| IBIS file usslh4gxxac.ibs
| 4Gb DDR3L SDRAM - Die Revision "D"
| This Model is valid for Commercial Temperature Range -40C<=Tc<=95C
| Valid for DDR3L-1066/1333/1600/1866/2133 operation
| Part Number   VDD/VDDQ   Architecture   Package
| SCB13H4G800AF   1.35V/1.35V   512Meg x 8   78-Ball 7.5x10.6mm FBGA
| SCB13H4G800AF KGD 1.35V/1.35V   512Meg x 8   Bare Die
| SCB13H4G160AF   1.35V/1.35V   256Meg x 16  96-Ball 7.5x13.5mm FBGA
| SCB13H4G160AF KGD 1.35V/1.35V   256Meg x 16  Bare Die
[IBIS Ver]   4.2
[File Name]   usslh4gxxac.ibs
[Date]   12/20/2020
[File Rev]   1.2
[Source]   UniIC
[Notes]   Revision History:
   Rev 1.0: 01/23/2019
   - For VDD1.50V
   Rev 1.1: 12/12/2019
   - Change VDD level to 1.35V from 1.50V
   Rev 1.2: 12/20/2020
   - Change temp to -40C from 0C
   - update 95c data
[Disclaimer]  --
[Copyright]   Copyright 2020. UniIC All rights reserved.
| COMPONENT: SCB13H4G800AF (78-Ball FBGA, x8, 7.5mm X 10.6mm)
[Component]   SCB13H4G800AF
[Package Model] f25_4gd3_x8_78ball_pkg
[Manufacturer]  UniIC.
[Package]
|   typ   min   max
R_pkg   404m   282m   555m
L_pkg   1.730nH   1.139nH   2.492nH
C_pkg   0.438pF   0.389pF   0.762pF
[Pin]   signal_name  model_name   R_pin  L_pin   C_pin
A1   VSS   GND
A2   VDD   POWER
A3   NC   NC
A7   NF_TDQS#   NF_TDQS#   474m   1.870nH   0.560pF
A8   VSS   GND
A9   VDD   POWER
B1   VSS   GND
B2   VSSQ   GND
B3   DQ0   DQ   499m   1.667nH   0.564pF
B7   DM_TDQS   DM_TDQS   474m   1.582nH   0.537pF
B8   VSSQ   GND
B9   VDDQ   POWER
C1   VDDQ   POWER
C2   DQ2   DQ   555m   2.075nH   0.595pF
C3   DQS   DQS   476m   1.795nH   0.574pF
C7   DQ1   DQ   401m   1.399nH   0.540pF
C8   DQ3   DQ   504m   1.705nH   0.567pF
C9   VSSQ   GND
D1   VSSQ   GND
D2   DQ6   DQ   504m   1.669nH   0.567pF
D3   DQS#   DQS   480m   1.782nH   0.568pF
D7   VDD   POWER
D8   VSS   GND
D9   VSSQ   GND
E1   VREFDQ   POWER
E2   VDDQ   POWER
E3   DQ4   DQ   399m   1.300nH   0.528pF
E7   DQ7   DQ   393m   1.400nH   0.549pF
E8   DQ5   DQ   472m   1.522nH   0.557pF
E9   VDDQ   POWER
F1   NC   NC
F2   VSS   GND
F3   RAS#   INPUT   367m   1.644nH   0.431pF
F7   CK   CLKIN   346m   1.230nH   0.390pF
F8   VSS   GND
F9   NC   NC
G1   ODT   INPUT   496m   2.492nH   0.516pF
G2   VDD   POWER
G3   CAS#   INPUT   397m   1.998nH   0.417pF
G7   CK#   CLKIN   349m   1.428nH   0.397pF
G8   VDD   POWER
G9   CKE   INPUT   432m   2.140nH   0.438pF
H1   NC   NC
H2   CS#   INPUT   376m   1.890nH   0.414pF
H3   WE#   INPUT   397m   1.729nH   0.41pF
H7   A10   INPUT   306m   1.139nH   0.402pF
H8   ZQ   NC   394m   1.459nH   0.417pF
H9   NC   NC
J1   VSS   GND
J2   BA0   INPUT   379m   1.786nH   0.401pF
J3   BA2   INPUT   446m   1.959nH   0.417pF
J7   A15   INPUT   282m   1.236nH   0.413pF
J8   VREFCA   POWER
J9   VSS   GND
K1   VDD   POWER
K2   A3   INPUT   404m   1.842nH   0.427pF
K3   A0   INPUT   323m   1.426nH   0.396pF
K7   A12   INPUT   319m   1.369nH   0.389pF
K8   BA1   INPUT   418m   1.866nH   0.445pF
K9   VDD   POWER
L1   VSS   GND
L2   A5   INPUT   394m   1.951nH   0.419pF
L3   A2   INPUT   336m   1.617nH   0.394pF
L7   A1   INPUT   310m   1.445nH   0.433pF
L8   A4   INPUT   405m   1.730nH   0.422pF
L9   VSS   GND
M1   VDD   POWER
M2   A7   INPUT   426m   2.163nH   0.456pF
M3   A9   INPUT   367m   1.851nH   0.433pF
M7   A11   INPUT   389m   1.709nH   0.415pF
M8   A6   INPUT   442m   2.110nH   0.458pF
M9   VDD   POWER
N1   VSS   GND
N2   RESET#   RESET   542m   1.964nH   0.762pF
N3   A13   INPUT   424m   2.205nH   0.441pF
N7   A14   INPUT   446m   1.873nH   0.447pF
N8   A8   INPUT   493m   2.378nH   0.503pF
N9   VSS   GND
|***********************PIN MAPPING*****************************************
[Pin Mapping] pulldown_ref pullup_ref gnd_clamp_ref power_clamp_ref ext_ref
A1   VSS   NC
A2   NC   VDD
A3   NC   NC
A7   VSS   VDDQ   VSS   VDDQ
A8   VSS   NC
A9   NC   VDD
B1   VSS   NC
B2   VSS   NC
B3   VSS   VDDQ   VSS   VDDQ
B7   VSS   VDDQ   VSS   VDDQ
B8   VSS   NC
B9   NC   VDDQ
C1   NC   VDDQ
C2   VSS   VDDQ   VSS   VDDQ
C3   VSS   VDDQ   VSS   VDDQ
C7   VSS   VDDQ   VSS   VDDQ
C8   VSS   VDDQ   VSS   VDDQ
C9   VSS   NC
D1   VSS   NC
D2   VSS   VDDQ   VSS   VDDQ
D3   VSS   VDDQ   VSS   VDDQ
D7   NC   VDD
D8   VSS   NC
D9   VSS   NC
E1   NC   VREFDQ
E2   NC   VDDQ
E3   VSS   VDDQ   VSS   VDDQ
E7   VSS   VDDQ   VSS   VDDQ
E8   VSS   VDDQ   VSS   VDDQ
E9   NC   VDDQ
F1   NC   NC
F2   VSSL   NC
F3   NC   NC   VSS   VDD
F7   NC   NC   VSS   VDD
F8   VSS   NC
F9   NC   NC
G1   NC   NC   VSS   VDD
G2   NC   VDDL
G3   NC   NC   VSS   VDD
G7   NC   NC   VSS   VDD
G8   NC   VDD
G9   NC   NC   VSS   VDD
H1   NC   NC
H2   NC   NC   VSS   VDD
H3   NC   NC   VSS   VDD
H7   NC   NC   VSS   VDD
H8   NC   NC
H9   NC   NC
J1   VSS   NC
J2   NC   NC   VSS   VDD
J3   NC   NC   VSS   VDD
J7   NC   NC   VSS   VDD
J8   NC   VREFCA
J9   VSS   NC
K1   NC   VDD
K2   NC   NC   VSS   VDD
K3   NC   NC   VSS   VDD
K7   NC   NC   VSS   VDD
K8   NC   NC   VSS   VDD
K9   NC   VDD
L1   VSS   NC
L2   NC   NC   VSS   VDD
L3   NC   NC   VSS   VDD
L7   NC   NC   VSS   VDD
L8   NC   NC   VSS   VDD
L9   VSS   NC
M1   NC   VDD
M2   NC   NC   VSS   VDD
M3   NC   NC   VSS   VDD
M7   NC   NC   VSS   VDD
M8   NC   NC   VSS   VDD
M9   NC   VDD
N1   VSS   NC
N2   NC   NC   VSS   VDD
N3   NC   NC   VSS   VDD
N7   NC   NC   VSS   VDD
N8   NC   NC   VSS   VDD
N9   VSS   NC
|**********************DIFF PIN*********************************************
[Diff_pin]   inv_pin   vdiff   tdelay_typ   tdelay_min   tdelay_max
   C3   D3   0.320V   0ns   NA   NA
   F7   G7   0.320V   0ns   NA   NA
| COMPONENT: SCB13H4G160AF (96-Ball FBGA, x16, 7.5mm X 13.5mm)
[Component]   SCB13H4G160AF
[Package Model] f25_4gd3_x16_96ball_pkg
[Manufacturer]  UniIC.
[Package]
|   typ   min   max
R_pkg   449m   320m   623m
L_pkg   1.828nH   1.147nH   3.053nH
C_pkg   0.538pF   0.376pF   0.812pF
[Pin]   signal_name  model_name   R_pin   L_pin   C_pin
A1   VDDQ   POWER
A2   DQ13   DQ   581m   2.212nH  0.592pF
A3   DQ15   DQ   536m   1.891nH  0.554pF
A7   DQ12   DQ   536m   1.903nH  0.565pF
A8   VDDQ   POWER
A9   VSS   GND
B1   VSSQ   GND
B2   VDD   POWER
B3   VSS   GND
B7   UDQS#   DQS   503m   1.737nH  0.583pF
B8   DQ14   DQ   582m   2.266nH  0.574pF
B9   VSSQ   GND
C1   VDDQ   POWER
C2   DQ11   DQ   488m   1.893nH  0.538pF
C3   DQ9   DQ   421m   1.377nH  0.561pF
C7   UDQS   DQS   507m   1.684nH  0.57pF
C8   DQ10   DQ   562m   2.137nH  0.556pF
C9   VDDQ   POWER
D1   VSSQ   GND
D2   VDDQ   POWER
D3   UDM   DM   424m   1.243nH  0.563pF
D7   DQ8   DQ   367m   1.215nH  0.531pF
D8   VSSQ   GND
D9   VDD   POWER
E1   VSS   GND
E2   VSSQ   GND
E3   DQ0   DQ   385m   1.248nH  0.558pF
E7   LDM   DM   384m   1.183nH  0.556pF
E8   VSSQ   GND
E9   VDDQ   POWER
F1   VDDQ   POWER
F2   DQ2   DQ   486m   1.450nH  0.569pF
F3   LDQS   DQS   441m   1.603nH  0.55pF
F7   DQ1   DQ   358m   1.147nH  0.544pF
F8   DQ3   DQ   454m   1.411nH  0.551pF
F9   VSSQ   GND
G1   VSSQ   GND
G2   DQ6   DQ   440m   1.316nH  0.541pF
G3   LDQS#   DQS   438m   1.640nH  0.542pF
G7   VDD   POWER
G8   VSS   GND
G9   VSSQ   GND
H1   VREFDQ   POWER
H2   VDDQ   POWER
H3   DQ4   DQ   402m   1.262nH  0.562pF
H7   DQ7   DQ   415m   1.353nH  0.563pF
H8   DQ5   DQ   544m   1.670nH  0.569pF
H9   VDDQ   POWER
J1   NC   NC
J2   VSS   GND
J3   RAS#   INPUT   320m   1.391nH  0.443pF
J7   CK   CLKIN   335m   1.168nH  0.376pF
J8   VSS   GND
J9   NC   NC
K1   ODT   INPUT   449m   2.344nH  0.449pF
K2   VDD   POWER
K3   CAS#   INPUT   328m   1.520nH  0.451pF
K7   CK#   CLKIN   327m   1.315nH  0.387pF
K8   VDD   POWER
K9   CKE   INPUT   496m   2.272nH  0.497pF
L1   NC   NC
L2   CS#   INPUT   414m   2.027nH  0.446pF
L3   WE#   INPUT   349m   1.670nH  0.436pF
L7   A10   INPUT   350m   1.335nH  0.447pF
L8   ZQ   NC   479m   1.675nH  0.492pF
L9   NC   NC
M1   VSS   GND
M2   BA0   INPUT   430m   2.210nH  0.443pF
M3   BA2   INPUT   400m   1.828nH  0.449pF
M7   NC   NC
M8   VREFCA   POWER
M9   VSS   GND
N1   VDD   POWER
N2   A3   INPUT   488m   2.298nH  0.493pF
N3   A0   INPUT   392m   1.664nH  0.456pF
N7   A12   INPUT   382m   1.894nH  0.476pF
N8   BA1   INPUT   484m   2.159nH  0.499pF
N9   VDD   POWER
P1   VSS   GND
P2   A5   INPUT   515m   2.412nH  0.524pF
P3   A2   INPUT   447m   2.102nH  0.537pF
P7   A1   INPUT   415m   2.085nH  0.516pF
P8   A4   INPUT   498m   2.422nH  0.534pF
P9   VSS   GND
R1   VDD   POWER
R2   A7   INPUT   565m   2.745nH  0.585pF
R3   A9   INPUT   492m   2.376nH  0.531pF
R7   A11   INPUT   452m   2.341nH  0.506pF
R8   A6   INPUT   559m   2.746nH  0.595pF
R9   VDD   POWER
T1   VSS   GND
T2   RESET#   RESET   623m   2.039nH  0.812pF
T3   A13   INPUT   556m   2.572nH  0.547pF
T7   A14   INPUT   518m   2.557nH  0.521pF
T8   A8   INPUT   583m   3.053nH  0.578pF
T9   VSS   GND
|***********************PIN MAPPING*****************************************
[Pin Mapping] pulldown_ref pullup_ref gnd_clamp_ref power_clamp_ref ext_ref
A1   NC   VDDQ
A2   VSS   VDDQ   VSS   VDDQ
A3   VSS   VDDQ   VSS   VDDQ
A7   VSS   VDDQ   VSS   VDDQ
A8   NC   VDDQ
A9   VSS   NC
B1   VSS   NC
B2   NC   VDD
B3   VSS   NC
B7   VSS   VDDQ   VSS   VDDQ
B8   VSS   VDDQ   VSS   VDDQ
B9   VSS   NC
C1   NC   VDDQ
C2   VSS   VDDQ   VSS   VDDQ
C3   VSS   VDDQ   VSS   VDDQ
C7   VSS   VDDQ   VSS   VDDQ
C8   VSS   VDDQ   VSS   VDDQ
C9   NC   VDDQ
D1   VSS   NC
D2   NC   VDDQ
D3   NC   NC   VSS   VDDQ
D7   VSS   VDDQ   VSS   VDDQ
D8   VSS   NC
D9   NC   VDD
E1   VSS   NC
E2   VSS   NC
E3   VSS   VDDQ   VSS   VDDQ
E7   NC   NC   VSS   VDDQ
E8   VSS   NC
E9   NC   VDDQ
F1   NC   VDDQ
F2   VSS   VDDQ   VSS   VDDQ
F3   VSS   VDDQ   VSS   VDDQ
F7   VSS   VDDQ   VSS   VDDQ
F8   VSS   VDDQ   VSS   VDDQ
F9   VSS   NC
G1   VSS   NC
G2   VSS   VDDQ   VSS   VDDQ
G3   VSS   VDDQ   VSS   VDDQ
G7   NC   VDD
G8   VSS   NC
G9   VSS   NC
H1   NC   VREFDQ
H2   NC   VDDQ
H3   VSS   VDDQ   VSS   VDDQ
H7   VSS   VDDQ   VSS   VDDQ
H8   VSS   VDDQ   VSS   VDDQ
H9   NC   VDDQ
J1   NC   NC
J2   VSSL   NC
J3   NC   NC   VSS   VDD
J7   NC   NC   VSS   VDD
J8   VSS   NC
J9   NC   NC
K1   NC   NC   VSS   VDD
K2   NC   VDDL
K3   NC   NC   VSS   VDD
K7   NC   NC   VSS   VDD
K8   NC   VDD
K9   NC   NC   VSS   VDD
L1   NC   NC
L2   NC   NC   VSS   VDD
L3   NC   NC   VSS   VDD
L7   NC   NC   VSS   VDD
L8   NC   NC
L9   NC   NC
M1   VSS   NC
M2   NC   NC   VSS   VDD
M3   NC   NC   VSS   VDD
M7   NC   NC
M8   NC   VREFCA
M9   VSS   NC
N1   NC   VDD
N2   NC   NC   VSS   VDD
N3   NC   NC   VSS   VDD
N7   NC   NC   VSS   VDD
N8   NC   NC   VSS   VDD
N9   NC   VDD
P1   VSS   NC
P2   NC   NC   VSS   VDD
P3   NC   NC   VSS   VDD
P7   NC   NC   VSS   VDD
P8   NC   NC   VSS   VDD
P9   VSS   NC
R1   NC   VDD
R2   NC   NC   VSS   VDD
R3   NC   NC   VSS   VDD
R7   NC   NC   VSS   VDD
R8   NC   NC   VSS   VDD
R9   NC   VDD
T1   VSS   NC
T2   NC   NC   VSS   VDD
T3   NC   NC   VSS   VDD
T7   NC   NC   VSS   VDD
T8   NC   NC   VSS   VDD
T9   VSS   NC
|**********************DIFF PIN*********************************************
[Diff_pin]   inv_pin   vdiff   tdelay_typ   tdelay_min   tdelay_max
   C7   B7   0.320V   0ns   NA   NA
   F3   G3   0.320V   0ns   NA   NA
   J7   K7   0.320V   0ns   NA   NA
| COMPONENT: SCB13H4G800AF KGD (Bare Die, x8)
[Component]   SCB13H4G800AF KGD
[Manufacturer]  UniIC.
[Package]
|   typ   min   max
R_pkg   0.001m   0.001m   0.001m
L_pkg   0.001nH   0.001nH   0.001nH
C_pkg   0.001pF   0.001pF   0.001pF
[Pin]   signal_name  model_name   R_pin   L_pin   C_pin
1   DNU   NC
2   VSS   GND
3   VDD   POWER
4   VDD   POWER
5   DNU   NC
6   VSS   GND
7   DNU   NC
8   VDDQ   POWER
9   DNU   NC
10   VSS   GND
11   DNU   NC
12   VDDQ   POWER
13   DNU   NC
14   VSS   GND
15   DNU   NC
16   DNU   NC
17   VDDQ   POWER
18   DNU   NC
19   VSS   GND
20   DNU   NC
21   VDDQ   POWER
22   DNU   NC
23   VSS   GND
24   DNU   NC
25   VDDQ   POWER
26   NF_TDQS#   NF_TDQS#
27   VSS   GND
28   VDD   POWER
29   VSS   GND
30   DM_TDQS   DM_TDQS
31   VDDQ   POWER
32   DQ0   DQ
33   VSS   GND
34   DQ1   DQ
35   VDDQ   POWER
36   DQ2   DQ
37   VSS   GND
38   DQ3   DQ
39   VDDQ   POWER
40   DQS   DQS
41   DQS#   DQS
42   VSS   GND
43   DQ6   DQ
44   VDDQ   POWER
45   DQ5   DQ
46   VSS   GND
47   DQ4   DQ
48   VDDQ   POWER
49   DQ7   DQ
50   VSS   GND
51   VREFDQ   POWER
52   VSS   GND
53   VDD   POWER
54   DNU   NC
55   VDD   POWER
56   VSS   GND
57   CK   CLKIN
58   CK#   CLKIN
59   CKE   INPUT
60   RAS#   INPUT
61   ODT   INPUT
62   CAS#   INPUT
63   CS#   INPUT
64   WE#   INPUT
65   A10   INPUT
66   VDD   POWER
67   VREFCA   POWER
68   VSS   GND
69   ZQ   NC
70   BA0   INPUT
71   BA1   INPUT
72   BA2   INPUT
73   A15   INPUT
74   A3   INPUT
75   A12   INPUT
76   VDD   POWER
77   VSS   GND
78   A0   INPUT
79   A4   INPUT
80   A5   INPUT
81   A6   INPUT
82   A2   INPUT
83   A1   INPUT
84   A7   INPUT
85   A8   INPUT
86   A9   INPUT
87   A11   INPUT
88   A13   INPUT
89   A14   INPUT
90   VDD   POWER
91   VSS   GND
92   RESET#   RESET
93   DNU   NC
94   DNU   NC
95   DNU   NC
96   DNU   NC
97   DNU   NC
98   DNU   NC
99   DNU   NC
100   VDD   POWER
101   VDD   POWER
102   VSS   GND
103   DNU   NC
|**********************DIFF PIN*********************************************
[Diff_pin]   inv_pin   vdiff   tdelay_typ   tdelay_min   tdelay_max
   40   41   0.320V   0ns   NA   NA
   57   58   0.320V   0ns   NA   NA
| COMPONENT: SCB13H4G160AF KGD (Bare Die, x16)
[Component]   SCB13H4G160AF KGD
[Manufacturer]  UniIC.
[Package]
|   typ   min   max
R_pkg   0.001m   0.001m   0.001m
L_pkg   0.001nH   0.001nH   0.001nH
C_pkg   0.001pF   0.001pF   0.001pF
[Pin]   signal_name  model_name   R_pin   L_pin   C_pin
1   DNU   NC
2   VSS   GND
3   VDD   POWER
4   VDD   POWER
5   DNU   NC
6   VSS   GND
7   DQ12   DQ
8   VDDQ   POWER
9   DQ15   DQ
10   VSS   GND
11   DQ13   DQ
12   VDDQ   POWER
13   DQ14   DQ
14   VSS   GND
15   UDQS#   DQS
16   UDQS   DQS
17   VDDQ   POWER
18   DQ9   DQ
19   VSS   GND
20   DQ8   DQ
21   VDDQ   POWER
22   DQ11   DQ
23   VSS   GND
24   DQ10   DQ
25   VDDQ   POWER
26   UDM   DM
27   VSS   GND
28   VDD   POWER
29   VSS   GND
30   LDM   DM
31   VDDQ   POWER
32   DQ0   DQ
33   VSS   GND
34   DQ1   DQ
35   VDDQ   POWER
36   DQ2   DQ
37   VSS   GND
38   DQ3   DQ
39   VDDQ   POWER
40   LDQS   DQS
41   LDQS#   DQS
42   VSS   GND
43   DQ6   DQ
44   VDDQ   POWER
45   DQ5   DQ
46   VSS   GND
47   DQ4   DQ
48   VDDQ   POWER
49   DQ7   DQ
50   VSS   GND
51   VREFDQ   POWER
52   VSS   GND
53   VDD   POWER
54   DNU   NC
55   VDD   POWER
56   VSS   GND
57   CK   CLKIN
58   CK#   CLKIN
59   CKE   INPUT
60   RAS#   INPUT
61   ODT   INPUT
62   CAS#   INPUT
63   CS#   INPUT
64   WE#   INPUT
65   A10   INPUT
66   VDD   POWER
67   VREFCA   POWER
68   VSS   GND
69   ZQ   NC
70   BA0   INPUT
71   BA1   INPUT
72   BA2   INPUT
73   DNU   NC
74   A3   INPUT
75   A12   INPUT
76   VDD   POWER
77   VSS   GND
78   A0   INPUT
79   A4   INPUT
80   A5   INPUT
81   A6   INPUT
82   A2   INPUT
83   A1   INPUT
84   A7   INPUT
85   A8   INPUT
86   A9   INPUT
87   A11   INPUT
88   A13   INPUT
89   A14   INPUT
90   VDD   POWER
91   VSS   GND
92   RESET#   RESET
93   DNU   NC
94   DNU   NC
95   DNU   NC
96   DNU   NC
97   DNU   NC
98   DNU   NC
99   DNU   NC
100   VDD   POWER
101   VDD   POWER
102   VSS   GND
103   DNU   NC
|**********************DIFF PIN*********************************************
[Diff_pin]   inv_pin   vdiff   tdelay_typ   tdelay_min   tdelay_max
   16   15   0.320V   0ns   NA   NA
   40   41   0.320V   0ns   NA   NA
   57   58   0.320V   0ns   NA   NA
|   Model Selector
[Model Selector] DQ
DQ_34   34 Ohm Data I/O with no ODT, 800-2133Mbps
DQ_40   40 Ohm Data I/O with no ODT, 800-2133Mbps
DQ_IN_ODT20   Data Input with 20ohm ODT, 800-2133Mbps
DQ_IN_ODT30   Data Input with 30ohm ODT, 800-2133Mbps
DQ_IN_ODT40   Data Input with 40ohm ODT, 800-2133Mbps
DQ_IN_ODT60   Data Input with 60ohm ODT, 800-2133Mbps
DQ_IN_ODT120  Data Input with 120ohm ODT, 800-2133Mbps
[Model Selector] DQS
DQS_34   34 Ohm Data Strobe I/O with no ODT, 800-2133Mbps
DQS_40   40 Ohm Data Strobe I/O with no ODT, 800-2133Mbps
DQS_IN_ODT20  Data Strobe Input with 20ohm ODT, 800-2133Mbps
DQS_IN_ODT30  Data Strobe Input with 30ohm ODT, 800-2133Mbps
DQS_IN_ODT40  Data Strobe Input with 40ohm ODT, 800-2133Mbps
DQS_IN_ODT60  Data Strobe Input with 60ohm ODT, 800-2133Mbps
DQS_IN_ODT120 Data Strobe Input with 120ohm ODT, 800-2133Mbps
[Model Selector] DM
DM_INPUT   DM Input Model with no ODT, 800-2133Mbps
DM_ODT20   DM Input Model with 20ohm ODT, 800-2133Mbps
DM_ODT30   DM Input Model with 30ohm ODT, 800-2133Mbps
DM_ODT40   DM Input Model with 40ohm ODT, 800-2133Mbps
DM_ODT60   DM Input Model with 60ohm ODT, 800-2133Mbps
DM_ODT120   DM Input Model with 120ohm ODT, 800-2133Mbps
[Model Selector] DM_TDQS
DM_INPUT   DM Input Model with no ODT, 800-2133Mbps
DM_ODT20   DM Input Model with 20ohm ODT, 800-2133Mbps
DM_ODT30   DM Input Model with 30ohm ODT, 800-2133Mbps
DM_ODT40   DM Input Model with 40ohm ODT, 800-2133Mbps
DM_ODT60   DM Input Model with 60ohm ODT, 800-2133Mbps
DM_ODT120   DM Input Model with 120ohm ODT, 800-2133Mbps
TDQS_ODT20   TDQS Terminator Model with 20ohm ODT, 800-2133Mbps
TDQS_ODT30   TDQS Terminator Model with 30ohm ODT, 800-2133Mbps
TDQS_ODT40   TDQS Terminator Model with 40ohm ODT, 800-2133Mbps
TDQS_ODT60   TDQS Terminator Model with 60ohm ODT, 800-2133Mbps
TDQS_ODT120   TDQS Terminator Model with 120ohm ODT, 800-2133Mbps
[Model Selector] NF_TDQS#
NF_INPUT   Non-Functioning Terminator Model
TDQS_ODT20   TDQS Terminator Model with 20ohm ODT, 800-2133Mbps
TDQS_ODT30   TDQS Terminator Model with 30ohm ODT, 800-2133Mbps
TDQS_ODT40   TDQS Terminator Model with 40ohm ODT, 800-2133Mbps
TDQS_ODT60   TDQS Terminator Model with 60ohm ODT, 800-2133Mbps
TDQS_ODT120   TDQS Terminator Model with 120ohm ODT, 800-2133Mbps
| Sparse Matrix Package Model for 4g3d_78ball_pkg (x4/x8)
[Define Package Model]  f25_4gd3_x8_78ball_pkg
[Manufacturer]  UniIC.
[OEM]   UniIC.
[Description]  4G3D package model for 7.5mm x 10.6mm 78-Ball FBGA
[Number of Pins] 46
[Pin Numbers]
A1  | VSS
A2  | VDD
A7  | DMU
B3  | DQ0
B7  | DML
B9  | VDDQ
C2  | DQ2
C3  | DQS
C7  | DQ1
C8  | DQ3
D2  | DQ6
D3  | DQSB
E1  | VREF_DQ
E3  | DQ4
E7  | DQ7
E8  | DQ5
F3  | RASB
F7  | CK
G1  | ODT
G3  | CASB
G7  | CKB
G9  | CKE
H2  | CSB
H3  | WEB
H7  | A10
H8  | ZQ
J2  | BA0
J3  | BA2
J7  | A15
J8  | VREF_CA
K2  | A3
K3  | A0
K7  | A12
K8  | BA1
L2  | A5
L3  | A2
L7  | A1
L8  | A4
M2  | A7
M3  | A9
M7  | A11
M8  | A6
N2  | RESETB
N3  | A13
N7  | A14
N8  | A8
[Model Data]
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[End Model Data]
[End Package Model]|
| Sparse Matrix Package Model for 4G3D_96ball_pkg (x16)
[Define Package Model]  f25_4gd3_x16_96ball_pkg
[Manufacturer]  UniIC.
[OEM]   UniIC.
[Description]  4G3D package model for 7.5mm x 13.5mm 96-Ball FBGA
[Number of Pins] 57
[Pin Numbers]
A1  | VDDQ_SUBNET_000
A2  | DQU5
A3  | DQU7
A7  | DQU4
A8  | VDDQ_SUBNET_001
A9  | VSS
B2  | VDD
B7  | DQSUB
B8  | DQU6
C2  | DQU3
C3  | DQU1
C7  | DQSU
C8  | DQU2
D3  | DMU
D7  | DQU0
E3  | DQL0
E7  | DML
F2  | DQL2
F3  | DQSL
F7  | DQL1
F8  | DQL3
G2  | DQL6
G3  | DQSLB
H1  | VREFDQ
H3  | DQL4
H7  | DQL7
H8  | DQL5
J3  | RASB
J7  | CK
K1  | ODT
K3  | CASB
K7  | CKB
K9  | CKE
L2  | CSB
L3  | WEB
L7  | A10
L8  | ZQ
M2  | BA0
M3  | BA2
M7  | A15
M8  | VREFCA
N2  | A3
N3  | A0
N7  | A12
N8  | BA1
P2  | A5
P3  | A2
P7  | A1
P8  | A4
R2  | A7
R3  | A9
R7  | A11
R8  | A6
T2  | RESETB
T3  | A13
T7  | A14
T8  | A8
[Model Data]
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[End Model Data]
[End Package Model]
| Models and submodels in the file (29): DQ_34 (I/O), DQ_40 (I/O), DQ_IN_ODT20 (Input), DQ_IN_ODT30 (Input), DQ_IN_ODT40 (Input), DQ_IN_ODT60 (Input), DQ_IN_ODT120 (Input), DQS_34 (I/O), DQS_40 (I/O), DQS_IN_ODT20 (Input), DQS_IN_ODT30 (Input), DQS_IN_ODT40 (Input), DQS_IN_ODT60 (Input), DQS_IN_ODT120 (Input), DM_INPUT (Input), DM_ODT20 (Input), DM_ODT30 (Input), DM_ODT40 (Input), DM_ODT60 (Input), DM_ODT120 (Input), TDQS_ODT20 (Terminator), TDQS_ODT30 (Terminator), TDQS_ODT40 (Terminator), TDQS_ODT60 (Terminator), TDQS_ODT120 (Terminator), INPUT (Input), CLKIN (Input), RESET (Input), NF_INPUT (Terminator)
